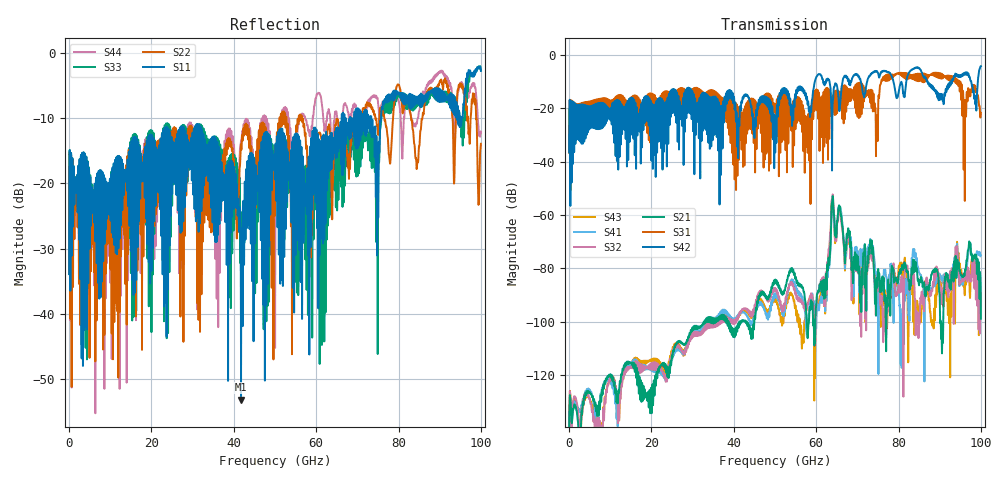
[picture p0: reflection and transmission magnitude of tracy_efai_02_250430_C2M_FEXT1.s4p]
!! PART DESCRIPTION: TE 224G+ VSR Channel- Chip to module, IO connector to CPC(Co-packaged connector) through over the board cable
!! CHANNEL DESCRIPTION: Module trace -> Mated IO 224G+ Connector -> Internal Cable Termination -> 30AWG 300mm Cable -> Cable
!!  termination + CPC connector(No footprint or package included)
!! MODEL REVISION:  Rev 3, Created on April 25, 2025
!! MODEL STATUS: Development
!! MODEL GEOMETRY: 8 Pair Channel
!! MODEL FREQUENCY RANGE: 0 GHz to 100 GHz in 10.00 MHz frequency steps
!! MODEL EDGE RATE LIMITATION: 5ps (Using conservative 0.5/Fmax rule of thumb)
!! PORT DEFINITIONS:
!! Port  1  ----->  Module Side  -->  Host Side, A Row  <-----  Port  2
!! Port  3  ----->  Module Side  -->  Host Side, A Row  <-----  Port  4
# GHz S MA R 45
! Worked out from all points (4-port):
!   10000 points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, 10 MHz to 100 GHz, reference 45 ohm
!   strongest paths, dB at 10 MHz, 25.01 GHz, 50.01 GHz, 75.01 GHz, 100 GHz:
!     S42: -36.5, -16.7, -29.8, -6.7, -4.3
!     S31: -36.7, -17.7, -20.3, -22.6, -21.7
!     S21: -140.7, -112.7, -84.6, -80.5, -98.8
!     S32: -142.0, -112.4, -87.6, -82.5, -89.3
!     S41: -142.9, -114.0, -89.6, -88.2, -75.0
!     S43: -143.0, -111.4, -91.2, -88.9, -91.9
!   lowest |S11| = -53.2 dB at 41.76 GHz (marker M1), VSWR 1.00, Z = 44.9 + j0.179 ohm
!   |S11| at or under -10 dB: start of sweep to 66.19 GHz; 67.15 GHz to 68.21 GHz (1.059 GHz wide, 1.57 % of centre); 73.39 GHz to 75.75 GHz (2.363 GHz wide, 3.17 % of centre)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
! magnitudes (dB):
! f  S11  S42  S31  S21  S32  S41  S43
! 10 MHz  -33.9  -36.5  -36.7  -140.7  -142.0  -142.9  -143.0
! 30.85 GHz  -16.6  -20.4  -16.1  -101.5  -103.9  -103.2  -103.7
! 41.76 GHz  -53.2  -18.8  -22.0  -100.0  -96.0  -96.4  -96.5
! 62.13 GHz  -12.9  -10.6  -13.3  -86.1  -85.7  -90.0  -90.7
! 64.01 GHz  -15.6  -17.7  -16.2  -52.9  -52.3  -54.5  -53.9
! 70.73 GHz  -12.2  -9.1  -16.5  -89.3  -100.6  -73.7  -78.0
! 100 GHz  -2.7  -4.3  -21.7  -98.8  -89.3  -75.0  -91.9
